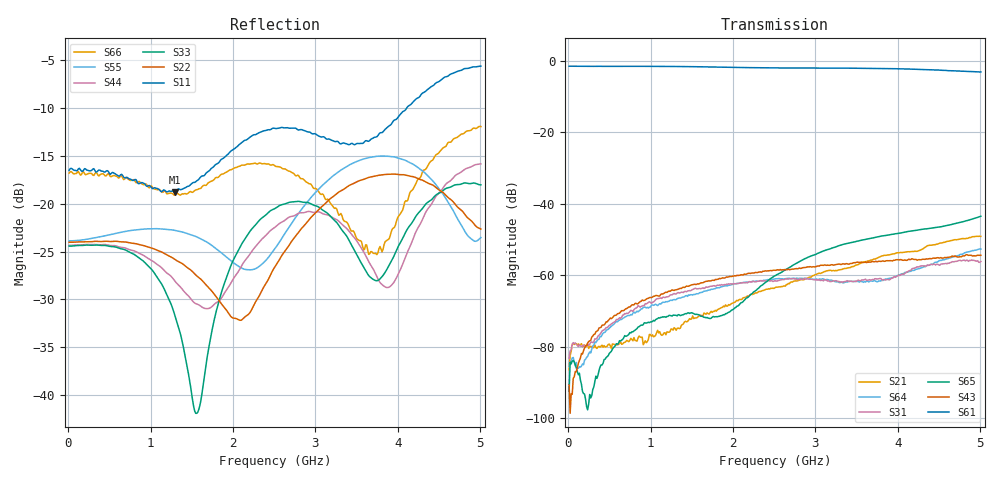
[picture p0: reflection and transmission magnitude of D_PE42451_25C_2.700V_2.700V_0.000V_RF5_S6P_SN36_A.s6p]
! Device ID: PE42451
! Serial: 36
! Insertion: A
! Temp: 25C
! VDD: 2.700
! Control_Hi: 100.000
! Control_Lo: 0.000
! Logic State: RF5
! Port 1: RFC
! Port 2: RF1
! Port 3: RF2
! Port 4: RF3
! Port 5: RF4
! Port 6: RF5
! V1 = 2.70
! V2 = 0.00
! V3 = 2.70
! V4 = 0.00
! IDD: 1.082380e-05
#  Hz  S  RI  R  50
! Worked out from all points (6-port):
!   401 points, 10 MHz to 5.01 GHz, reference 50 ohm
!   strongest paths, dB at 10 MHz, 1.26 GHz, 2.51 GHz, 3.76 GHz, 5.01 GHz:
!     S61: -1.6, -1.6, -2.0, -2.2, -3.2
!     S43: -90.7, -64.1, -58.6, -56.2, -54.4
!     S65: -92.5, -71.4, -60.1, -49.3, -43.5
!     S31: -83.2, -65.5, -61.5, -61.0, -56.2
!     S64: -85.5, -67.1, -61.0, -61.8, -52.7
!     S21: -86.5, -75.0, -63.5, -55.1, -49.1
!   lowest |S11| = -18.8 dB at 1.298 GHz (marker M1), VSWR 1.26, Z = 54.8 - j11.1 ohm
!   |S11| at or under -10 dB: start of sweep to 4.11 GHz
